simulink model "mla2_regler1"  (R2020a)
settings: Solver=ode5  StartTime=0.0  StopTime=0.3  FixedStep=0.0001  RelTol=1e-4  EnableMultiTasking=on
PreLoadFcn:
  | MLA_Sensor1 = load('mla_sensor1.dat');
libraries: libmla x1, simulink_need_slupdate x1

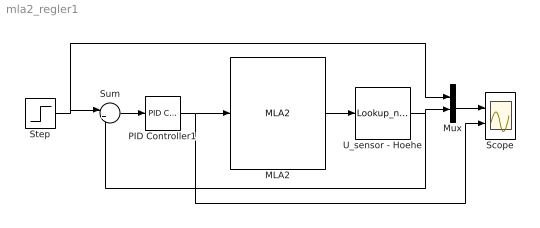
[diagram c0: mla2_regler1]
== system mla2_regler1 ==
  MLA2 : libmla/MLA2  g=9.81  m=0.125  Fr_g=0.14  Fr_h=0.16  d_l=0.18  d_t=0.1  a=40691  b=0.0687  N=4.282
  Mux : Mux  Inputs=2
  PID Controller1 : simulink_need_slupdate/PID Controller  P=7000  I=2000  D=50
  Scope : Scope  NumInputPorts=2
  Step : Step  Time=0.1  After=0.02  SampleTime=0
  Sum : Sum  Inputs=|+-
  U_sensor - Hoehe : Lookup_n-D  NumberOfTableDimensions=1  BreakpointsForDimension1=MLA_Sensor1(:,1)  Table=MLA_Sensor1(:,2)  RndMeth=Simplest
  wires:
  MLA2/1 -> U_sensor - Hoehe/1
  Mux/1 -> Scope/1
  Sum/1 -> PID Controller1/1
  Step/1 -> Sum/1, Mux/1
  U_sensor - Hoehe/1 -> Mux/2, Sum/2
  PID Controller1/1 -> MLA2/1, Scope/2
